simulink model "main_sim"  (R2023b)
settings: Solver=ode1  StartTime=0.0  StopTime=12  FixedStep=0.01  RelTol=1e-3

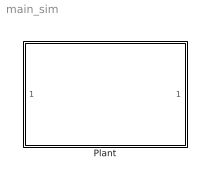
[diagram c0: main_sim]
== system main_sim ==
  Plant : Subsystem  TreatAsAtomicUnit=on  SystemSampleTime=0.01

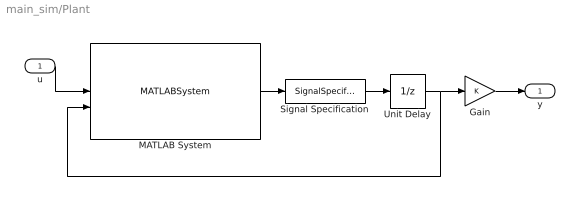
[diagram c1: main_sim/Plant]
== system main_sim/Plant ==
  u : Inport
  Gain : Gain  Multiplication=Matrix(K*u)
  MATLAB System : MATLABSystem  System=Plant  SimulateUsing=Code generation
  Signal Specification : SignalSpecification  Dimensions=[1, 1]
  Unit Delay : UnitDelay  SampleTime=-1  HasFrameUpgradeWarning=on
  y : Outport
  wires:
  u/1 -> MATLAB System/1
  MATLAB System/1 -> Signal Specification/1
  Signal Specification/1 -> Unit Delay/1
  Gain/1 -> y/1
  Unit Delay/1 -> Gain/1, MATLAB System/2
